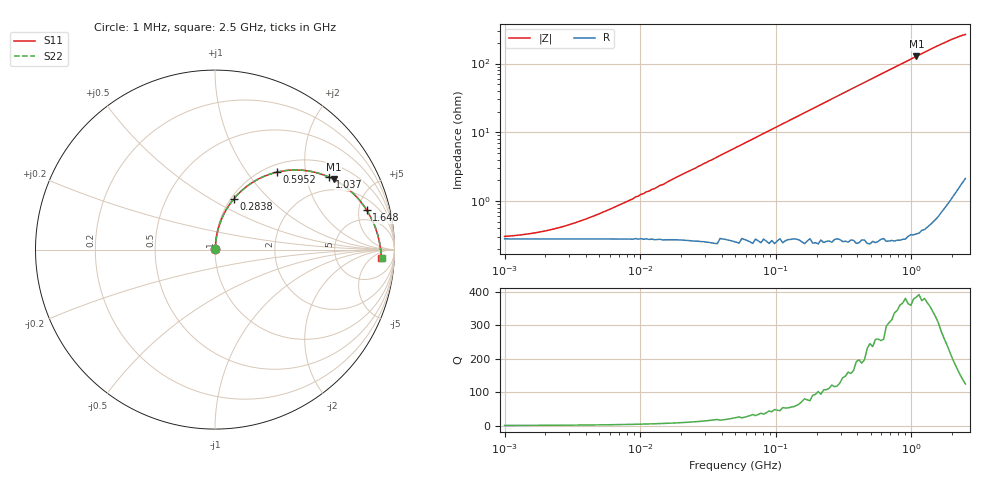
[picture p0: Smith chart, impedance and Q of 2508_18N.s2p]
# MHz S MA R 50
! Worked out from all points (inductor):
!   170 points, 1 MHz to 2.5 GHz, reference 50 ohm
!   read as one part in series: L = 18.8 nH near 7.321 MHz
!   highest Q = 385 at 1.086 GHz (marker M1), where L = 18.7 nH
!   S11 on the Smith chart (normalised r, x): 1 MHz: 1.01, +0.00; 283.8 MHz: 1.03, +0.64; 595.2 MHz: 1.13, +1.40; 1.037 GHz: 1.47, +2.74; 1.648 GHz: 3.30, +6.12; 2.5 GHz: 18, -13
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1  0.002838 22.9  0.997 -0.1  0.997 -0.1  0.002838 22.9
2.003  0.003427 40.2  0.997 -0.1  0.997 -0.1  0.003428 40.2
3.829  0.004981 58.1  0.997 -0.3  0.997 -0.3  0.004983 58.1
8.81  0.01 74.4  0.997 -0.6  0.997 -0.6  0.01 74.4
9.228  0.011 75.0  0.997 -0.7  0.997 -0.7  0.011 75.0
12.76  0.014 78.6  0.997 -0.9  0.997 -0.9  0.014 78.6
13.998  0.016 79.4  0.997 -1.0  0.997 -1.0  0.016 79.4
14.661  0.016 79.8  0.997 -1.0  0.997 -1.0  0.016 79.8
18.479  0.021 81.4  0.997 -1.3  0.997 -1.3  0.021 81.4
51.171  0.057 83.7  0.996 -3.7  0.996 -3.7  0.057 83.7
102.474  0.113 81.4  0.991 -7.3  0.991 -7.3  0.113 81.4
187.066  0.203 76.1  0.977 -13.2  0.977 -13.2  0.203 76.1
283.76  0.3 69.8  0.951 -19.8  0.951 -19.8  0.3 69.8
410.96  0.414 61.9  0.908 -27.8  0.908 -27.8  0.415 61.9
595.181  0.551 51.5  0.832 -38.3  0.832 -38.3  0.551 51.5
683.861  0.604 47.0  0.795 -42.8  0.795 -42.8  0.604 47.0
861.983  0.691 39.0  0.721 -50.8  0.721 -50.8  0.691 39.0
1037.345  0.754 32.3  0.654 -57.6  0.654 -57.6  0.755 32.3
1086.499  0.769 30.5  0.637 -59.3  0.637 -59.3  0.769 30.5
1648.104  0.874 14.5  0.482 -75.3  0.482 -75.3  0.874 14.5
2077.377  0.91 5.1  0.408 -84.5  0.408 -84.5  0.911 5.1
2500  0.928 -3.0  0.363 -92.5  0.363 -92.5  0.929 -3.0
